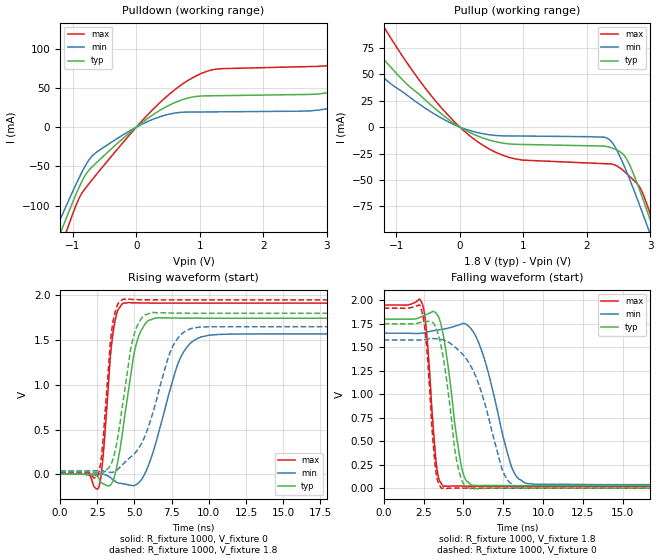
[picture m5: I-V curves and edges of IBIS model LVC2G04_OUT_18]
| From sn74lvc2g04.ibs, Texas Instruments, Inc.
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[Model]   LVC2G04_OUT_18
Model_type  Output
Vref =   0
Rref =   1000
Cref =   30p
Vmeas =   0.9
| variable   typ   min   max
C_comp   9.78pF   6.40pF   15.72pF
| C_pullup   9.15pF   6.40pF   10.43pF
| C_pulldown   10.40pF   6.59pF   15.72pF
[Temperature Range]   40   100   -40
| Ambient temperature   25   85   -40
[Voltage range]   1.8   1.65   1.95
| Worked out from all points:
|   slope of the pulldown table from 0 to 0.27 V, typ, clamps not added: 16.6 ohm
|   slope of the pullup table from 0 to 0.27 V, typ, clamps not added: 33 ohm
|   rising waveform, R_fixture 1000, V_fixture 0: 20-80 % time 942ps typ, 1.6ns min, 537ps max; typ from 0 V to 1.74 V
|   falling waveform, R_fixture 1000, V_fixture 1.8: 20-80 % time 809ps typ, 1.39ns min, 482ps max; typ from 1.8 V to 0.027 V
|   rising waveform, R_fixture 1000, V_fixture 1.8: 20-80 % time 958ps typ, 1.79ns min, 543ps max; typ from 0.027 V to 1.8 V
|   falling waveform, R_fixture 1000, V_fixture 0: 20-80 % time 796ps typ, 1.66ns min, 473ps max; typ from 1.75 V to 0 V
[Pulldown]
| LVC2G04_OUT_18
|   Voltage   I(typ)   I(min)   I(max)
-5.5V     -1.024A    -932.8mA   -1.143A
-1.25V    -145.7mA   -126.9mA   -167.2mA
-1.105V   -116mA     -100.2mA   -133.6mA
-650mV    -46.91mA   -33.3mA    -62.35mA
825mV     37.35mA    19.19mA    60.06mA
3.115V    45.49mA    25.17mA    79.66mA
3.755V    64.52mA    35.93mA    102.7mA
4.19V     79.14mA    21.53mA    128.2mA
4.47V     45.47mA    21.68mA    146.2mA
4.725V    44.49mA    21.83mA    131.7mA
5.01V     44.71mA    22mA       83.05mA
11V       50.72mA    25.33mA    92.94mA
[Pullup]
| LVC2G04_OUT_18
|   Voltage   I(typ)   I(min)   I(max)
-5.5V     449.7mA    254mA      638.5mA
-2.225V   143.3mA    107.6mA    207.3mA
-1.755V   105.1mA    78.04mA    153.5mA
-1.195V   63.95mA    46.44mA    94.81mA
-375mV    16.75mA    11.48mA    24.15mA
420mV     -11.47mA   -6.842mA   -19.31mA
2.34V     -18.76mA   -11.2mA    -34.79mA
2.645V    -32.43mA   -45.25mA   -45.19mA
2.84V     -61.19mA   -75.65mA   -57.82mA
2.99V     -86.8mA    -100.4mA   -81.09mA
3.08V     -102.8mA   -115.6mA   -97.77mA
11V       -1.709A    -1.61A     -1.847A
[Ramp]
| LVC2G04_OUT_18
| variable   typ   min   max
dV/dt_r   1.13/1.07E-09   1.02/1.77E-09   1.25/6.23E-10
dV/dt_f   1.11/9.00E-10   1.03/1.53E-09   1.20/5.13E-10
R_load = 1000
[Rising Waveform]
| LVC2G04_OUT_18
R_fixture =   1000
C_fixture =   0
L_fixture =   0
V_fixture =   0
V_fixture_min = 0
V_fixture_max = 0
|   Time   V(typ)   V(min)   V(max)
0s        112.7pV    7.663nV    3.037nV
2.605ns   -44.07mV   2.844mV    -142.7mV
2.885ns   -105.7mV   69.26uV    192.4mV
3.535ns   -80.96mV   -57.31mV   1.555V
4.245ns   527.8mV    -106.8mV   1.913V
4.965ns   1.345V     -126.6mV   1.917V
5.7ns     1.678V     6.504mV    1.915V
7.92ns    1.746V     1.235V     1.913V
9.28ns    1.745V     1.522V     1.913V
24.99ns   1.744V     1.569V     1.913V
[Falling Waveform]
| LVC2G04_OUT_18
R_fixture =   1000
C_fixture =   0
L_fixture =   0
V_fixture =   1.8
V_fixture_min = 1.65
V_fixture_max = 1.95
|   Time   V(typ)   V(min)   V(max)
0s        1.8V       1.65V      1.95V
2.44ns    1.831V     1.651V     1.951V
2.72ns    1.852V     1.661V     1.603V
3.295ns   1.86V      1.681V     265.4mV
3.75ns    1.619V     1.693V     20.88mV
4.875ns   228.7mV    1.747V     22.7mV
5.52ns    32.54mV    1.688V     21.24mV
8.015ns   27.52mV    230.3mV    21.07mV
8.84ns    27.2mV     59.22mV    21.09mV
24.99ns   26.98mV    37.16mV    21.09mV
[Rising Waveform]
| LVC2G04_OUT_18
R_fixture =   1000
C_fixture =   0
L_fixture =   0
V_fixture =   1.8
V_fixture_min = 1.65
V_fixture_max = 1.95
|   Time   V(typ)   V(min)   V(max)
0s        26.95mV    37.1mV     21.07mV
2.58ns    8.822mV    39.43mV    7.67mV
2.855ns   9.268mV    37.52mV    329.3mV
3.495ns   140.7mV    21.42mV    1.637V
4.215ns   794.8mV    111.3mV    1.955V
4.815ns   1.457V     202.4mV    1.954V
5.495ns   1.748V     350.2mV    1.952V
7.415ns   1.803V     1.371V     1.95V
8.675ns   1.8V       1.621V     1.95V
24.99ns   1.8V       1.65V      1.95V
[Falling Waveform]
| LVC2G04_OUT_18
R_fixture =   1000
C_fixture =   0
L_fixture =   0
V_fixture =   0
V_fixture_min = 0
V_fixture_max = 0
|   Time   V(typ)   V(min)   V(max)
0s        1.749V     1.578V     1.916V
2.34ns    1.766V     1.578V     1.914V
2.67ns    1.776V     1.586V     1.547V
3.24ns    1.721V     1.592V     222.8mV
3.645ns   1.474V     1.582V     -1.505mV
4.62ns    260.5mV    1.48V      1.404mV
5.435ns   -5.03mV    1.309V     32.61uV
7.415ns   290.6uV    208.5mV    -12.35uV
8.325ns   91.82uV    10.8mV     15.49uV
24.99ns   22.18uV    44.33uV    13.82uV
